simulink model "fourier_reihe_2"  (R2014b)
settings: Solver=ode45  StartTime=0.0  StopTime=10.0  RelTol=1e-3
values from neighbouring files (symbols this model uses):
  ampl1 = 1e-4    (= 0.0001)    [ad_test_2.m]    (also in ad_test_3.m; DA_wandler_spektr_1.m = 1; DA_wandler_spektr_2.m = 1; fourier_reihe1.m = 5)
  ampl2 = 1e-5    (= 1e-05)    [ad_test_2.m]    (also in ad_test_3.m; DA_wandler_spektr_1.m = 1; DA_wandler_spektr_2.m = 1; fourier_reihe1.m = 12)
  ampl3 = 6    [fourier_reihe1.m]    (also in fourier_reihe2.m; anti_alias_1.m = 0.2; anti_alias_2.m = 0.2; anti_alias_3.m = 0.2)
  f1 = 10    [DA_wandler_spektr_1.m]    (also in DA_wandler_spektr_2.m; fourier_reihe1.m = 100; fourier_reihe2.m = 100; mehrdeutigkeit_1.m = -200)
  f2 = 40    [DA_wandler_spektr_1.m]    (also in DA_wandler_spektr_2.m; fourier_reihe1.m = ',num2str(f2),     ' Hz; fourier_reihe2.m = 200; mehrdeutigkeit_1.m = 1800)
  f3 = ',num2str(f3),' Hz )']    [fourier_reihe1.m]    (also in fourier_reihe2.m = 2300; anti_alias_1.m = 250; anti_alias_2.m = 250; anti_alias_3.m = 250)
  fs = 4000    [abtast_rate_1.m]    (also in ad_test_12.m = ',     num2str(fs),'; ad_test_2.m = ',     num2str(fs),'; ad_test_3.m = ',     num2str(fs),'; DA_wandler_spektr_1.m = 100)
  N = 4*1024    (= 4096)    [ad_test_12.m]    (also in ad_test_2.m; ad_test_3.m; DA_wandler_spektr_1.m = 1000; DA_wandler_spektr_2.m = 1024)
  phi1 = pi/3    (= 1.0471975512)    [fourier_reihe1.m]    (also in fourier_reihe2.m; leakage_3.m; leakage_4.m; mehrdeutigkeit_1.m = 3.14159265359)
  phi2 = pi/4    (= 0.785398163397)    [fourier_reihe1.m]    (also in fourier_reihe2.m; leakage_3.m = 0.628318530718; leakage_4.m = 0.628318530718; mehrdeutigkeit_1.m = 3.14159265359)
  phi3 = -pi/5    (= -0.628318530718)    [fourier_reihe1.m]    (also in fourier_reihe2.m)
  xm = -10    [fourier_reihe1.m]    (also in fourier_reihe2.m; einseitig_1.m = xti.*xr - xtq.*xi)
undefined symbols (not defined in the file or in its folder): get
libraries: dsparch4 x2, dspspect3 x1, dspsnks4 x1

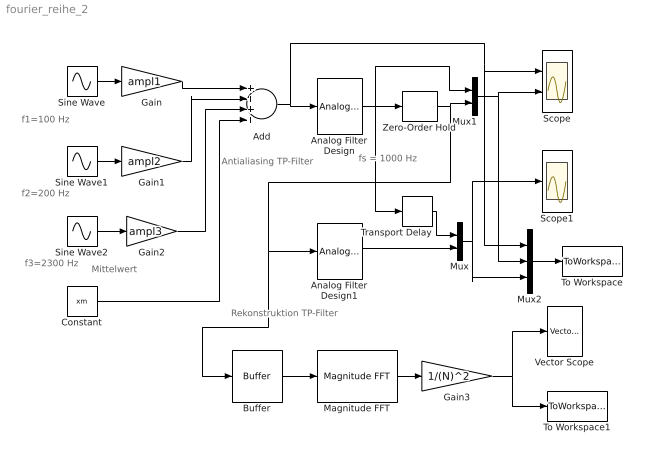
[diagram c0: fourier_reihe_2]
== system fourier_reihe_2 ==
  note: fs = 1000 Hz
  note: Rekonstruktion TP-Filter
  note: Antialiasing TP-Filter
  note: Mittelwert
  note: f3=2300 Hz
  note: f2=200 Hz
  note: f1=100 Hz
  Add : Sum  Inputs=++++
  Analog Filter Design : dsparch4/Analog Filter Design  method=Butterworth  filttype=Lowpass  N=8  Wlo=2*pi*fs/2  Whi=80  Rp=2  Rs=40
  Analog Filter Design1 : dsparch4/Analog Filter Design  method=Butterworth  filttype=Lowpass  N=8  Wlo=2*pi*fs/2  Whi=80  Rp=2  Rs=40
  Buffer : Buffer  N=N  TreatMby1Signals=One channel
  Constant : Constant  Value=xm
  Gain : Gain  Gain=ampl1
  Gain1 : Gain  Gain=ampl2
  Gain2 : Gain  Gain=ampl3
  Gain3 : Gain  Gain=1/(N)^2
  Magnitude FFT : dspspect3/Magnitude FFT  mag_or_magsq=Magnitude squared  FFTImplementation=Auto  fftLenInherit=on  fftsize=256  WrapInput=on
  Mux : Mux  Inputs=2
  Mux1 : Mux  Inputs=2
  Mux2 : Mux  Inputs=3
  Scope : Scope  NumInputPorts=2
  Scope1 : Scope
  Sine Wave : Sin  Frequency=2*pi*f1  Phase=phi1  SampleTime=0
  Sine Wave1 : Sin  Frequency=2*pi*f2  Phase=phi2  SampleTime=0
  Sine Wave2 : Sin  Frequency=2*pi*f3  Phase=phi3  SampleTime=0
  To Workspace : ToWorkspace  VariableName=y  SaveFormat=Structure With Time  SampleTime=-1
  To Workspace1 : ToWorkspace  VariableName=P  SampleTime=-1
  Transport Delay : TransportDelay  DelayTime=0.0022
  Vector Scope : dspsnks4/Vector Scope  ScopeProperties=on  Domain=Frequency  HorizSpan=1  DisplayProperties=off  AxisGrid=on  Memory=off  FrameNumber=on  AxisLegend=off  AxisZoom=off  OpenScopeAtSimStart=on  OpenScopeImmediately=off  FigPos=get(0,'defaultfigureposition')  AxisProperties=off  XUnits=Hertz  XRange=[0...Fs]  InheritXIncr=off  XIncr=Ts  XLabel=Time  XLimit=Auto  XMin=0  XMax=1  XStart=0  YUnits=dB  YLabel=Leistung in dB  LineProperties=off  XAxisParamsVer=6.9
  Zero-Order Hold : ZeroOrderHold  SampleTime=1/fs
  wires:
  Sine Wave/1 -> Gain/1
  Sine Wave2/1 -> Gain2/1
  Gain/1 -> Add/1
  Sine Wave1/1 -> Gain1/1
  Gain2/1 -> Add/3
  Analog Filter Design/1 -> Mux1/1, Transport Delay/1, Zero-Order Hold/1
  Add/1 -> Mux2/1, Scope/1, Analog Filter Design/1
  Zero-Order Hold/1 -> Buffer/1, Analog Filter Design1/1, Mux1/2
  Gain1/1 -> Add/2
  Constant/1 -> Add/4
  Analog Filter Design1/1 -> Mux/2
  Transport Delay/1 -> Mux/1
  Mux1/1 -> Mux2/2, Scope/2
  Mux/1 -> Mux2/3, Scope1/1
  Mux2/1 -> To Workspace/1
  Magnitude FFT/1 -> Gain3/1
  Gain3/1 -> To Workspace1/1, Vector Scope/1
  Buffer/1 -> Magnitude FFT/1
